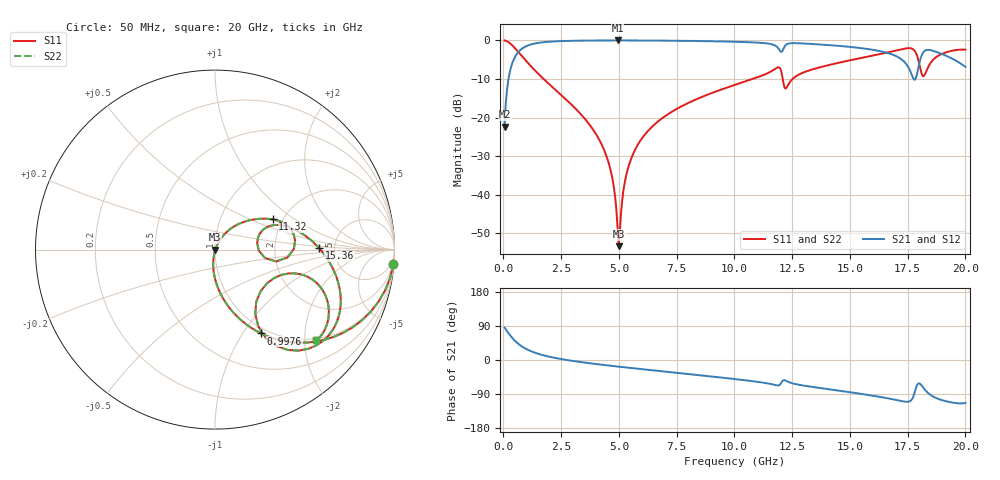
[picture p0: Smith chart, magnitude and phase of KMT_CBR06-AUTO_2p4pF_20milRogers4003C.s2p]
! Data measured by Modelithics Inc. support@modelithics.com 813-866-6335
! KEMET CBR06-AUTO 2.4pF, Pad Width= 0.851mm, Pad Length= 0.64mm, Pad Gap= 0.62mm, 20mil Rogers 4003C substrate Data, January 2022
# hz S ma R 50
! 2 Port Network Data from SP1.SP block
! freq  magS11  angS11  magS21  angS21  magS12  angS12  magS22  angS22
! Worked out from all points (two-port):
!   401 points, 50 MHz to 20 GHz, reference 50 ohm
!   highest |S21| = -0.02 dB at 4.938 GHz (marker M1); lowest = -22.4 dB at 50 MHz (marker M2)
!   |S21| within 3 dB of the highest: 644.6 MHz to 16.48 GHz (15.83 GHz wide, 185 % of centre); 18.19 GHz to 18.76 GHz (571.8 MHz wide, 3.09 % of centre)
!   lowest |S11| = -53.3 dB at 4.988 GHz (marker M3), VSWR 1.00, Z = 50.2 - j0.105 ohm
!   |S11| at or under -10 dB: 1.74 GHz to 10.79 GHz (9.049 GHz wide, 144 % of centre); 12.09 GHz to 12.52 GHz (424.3 MHz wide, 3.45 % of centre)
!   |S22| runs from -53.3 to 0.0 dB; largest |S21 - S12| = 0
!   S11 on the Smith chart (normalised r, x): 50 MHz: 1, -25; 997.6 MHz: 0.93, -1.21; 11.32 GHz: 1.78, +0.69; 15.36 GHz: 3.78, +0.08; 20 GHz: 0.96, -2.27
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5e7  0.9971 -4.5  0.07616 85.4  0.07616 85.4  0.9971 -4.5
3.4925e8  0.881 -29.4  0.4721 60.5  0.4721 60.5  0.881 -29.4
9.97625e8  0.5337 -61.1  0.8444 28.7  0.8444 28.7  0.5337 -61.1
3.391625e9  0.1071 -94.9  0.9923 -5.8  0.9923 -5.8  0.1071 -94.9
4.488875e9  0.02992 -100.2  0.9974 -14.1  0.9974 -14.1  0.02992 -100.2
4.73825e9  0.01498 -97.9  0.9976 -15.9  0.9976 -15.9  0.01498 -97.9
4.93775e9  0.003891 -74.4  0.9977 -17.2  0.9977 -17.2  0.003891 -74.4
4.987625e9  0.002162 -29.0  0.9977 -17.6  0.9977 -17.6  0.002162 -29.0
5.286875e9  0.01637 62.8  0.9975 -19.6  0.9975 -19.6  0.01637 62.8
5.53625e9  0.02976 64.5  0.9971 -21.2  0.9971 -21.2  0.02976 64.5
6.73325e9  0.09113 59.6  0.9931 -28.9  0.9931 -28.9  0.09113 59.6
1.0025e10  0.2654 38.8  0.9598 -50.3  0.9598 -50.3  0.2654 38.8
1.132175e10  0.3627 27.7  0.9205 -60.6  0.9205 -60.6  0.3627 27.7
1.206988e10  0.3467 -11.0  0.7239 -56.0  0.7239 -56.0  0.3467 -11.0
1.226938e10  0.2477 15.2  0.8918 -56.0  0.8918 -56.0  0.2477 15.2
1.336662e10  0.42 17.8  0.8979 -70.9  0.8979 -70.9  0.42 17.8
1.536162e10  0.5815 0.7  0.8014 -88.2  0.8014 -88.2  0.5815 0.7
1.670825e10  0.7065 -14.4  0.6761 -101.9  0.6761 -101.9  0.7065 -14.4
1.775562e10  0.7595 -46.6  0.3172 -94.8  0.3172 -94.8  0.7595 -46.6
1.805488e10  0.423 -58.0  0.5776 -63.7  0.5776 -63.7  0.423 -58.0
1.845388e10  0.4891 -16.1  0.7509 -90.7  0.7509 -90.7  0.4891 -16.1
2e10  0.7582 -41.8  0.4547 -113.5  0.4547 -113.5  0.7582 -41.8
